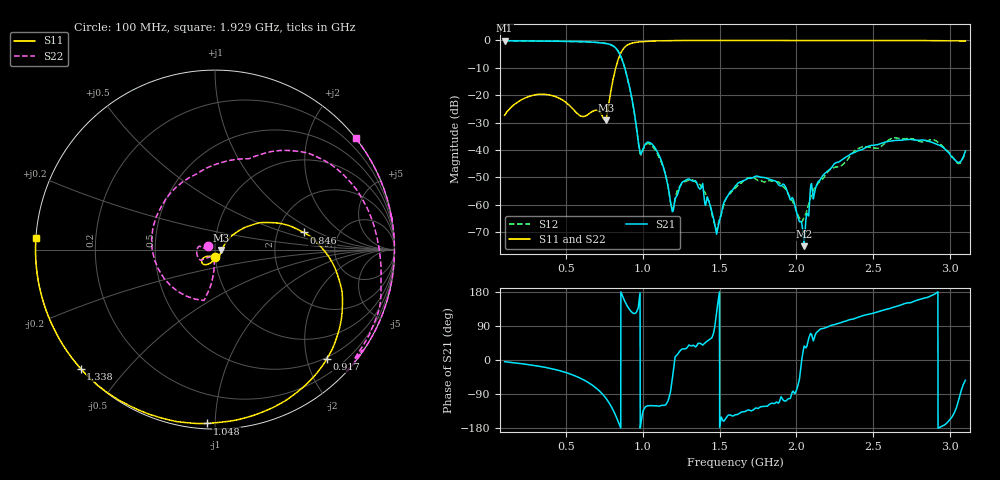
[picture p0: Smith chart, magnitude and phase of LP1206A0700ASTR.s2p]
!	AVX THIN FILM OPERATION
!	LP1206 High Performance Low Pass Filters
!	P/N LP1206A0700ASTR  4 September 2018
!Instrument: 	"HEWLETT PACKARD,8720ES,US39172150,7.62 "
! Created Tue Sep 04 12:40:53 2018
# MHz S db R 50
! freq  dbS11  angS11  dbS21  angS21  dbS12  angS12  dbS22  angS22
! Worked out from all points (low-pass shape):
!   3001 points, 100 MHz to 3.1 GHz, reference 50 ohm
!   highest |S21| = -0.09 dB at 100 MHz (marker M1); lowest = -75.1 dB at 2.05 GHz (marker M2)
!   |S21| within 3 dB of the highest: start of sweep to 828.3 MHz
!   lowest |S11| = -29.2 dB at 760 MHz (marker M3), VSWR 1.07, Z = 53.6 - j0.251 ohm
!   |S11| at or under -10 dB: start of sweep to 823.6 MHz
!   |S22| runs from -29.2 to 0.0 dB; largest |S21 - S12| = 0.024
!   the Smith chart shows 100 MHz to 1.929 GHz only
!   S11 on the Smith chart (normalised r, x): 100 MHz: 1.00, -0.09; 846 MHz: 2.81, +0.72; 917 MHz: 0.47, -2.37; 1.048 GHz: 0.03, -0.95; 1.338 GHz: 0.00, -0.38; 1.929 GHz: -0.00, +0.03
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100  -27.34 -88.4  -0.09 -4.5  -0.09 -4.4  -27.34 153.5
344  -19.63 -131.4  -0.22 -17.9  -0.29 -18.0  -19.63 -158.7
600  -27.69 -112.6  -0.45 -49.4  -0.40 -49.0  -27.69 -111.9
760  -29.17 -3.9  -1.09 -101.0  -1.03 -101.0  -29.17 -94.0
813  -12.48 34.4  -2.26 -137.6  -2.28 -138.1  -12.48 -99.2
846  -5.97 11.0  -4.60 -169.1  -4.52 -171.2  -5.97 80.8
917  -1.20 -44.4  -17.97 131.1  -18.17 131.3  -1.20 17.7
982  -0.51 -73.7  -40.92 177.5  -41.35 -175.0  -0.51 -11.2
1048  -0.27 -92.7  -37.35 -120.3  -37.91 -121.6  -0.27 -18.4
1100  -0.15 -104.2  -41.31 -121.8  -42.02 -122.7  -0.15 -31.9
1191  -0.07 -119.8  -62.22 -52.7  -61.38 -41.0  -0.07 -35.4
1260  -0.02 -129.3  -51.62 29.3  -51.98 34.1  -0.02 -38.1
1338  0.00 -138.5  -51.31 36.2  -51.42 40.0  0.00 -40.9
1481  0.00 -152.3  -70.48 129.5  -69.15 150.0  0.00 -28.6
1600  0.00 -162.1  -53.32 -144.6  -54.08 -138.5  0.00 -18.4
1929  0.00 176.2  -53.49 -108.4  -54.25 -100.0  -0.00 38.3
2050  0.00 169.3  -75.14 37.0  -64.51 44.8  0.00 55.6
2100  0.00 166.4  -53.12 65.3  -56.14 70.2  0.00 68.7
2368  0.00 152.3  -41.07 107.9  -41.02 111.5  0.00 120.5
2600  -0.00 140.5  -36.85 135.0  -36.38 140.2  0.00 -178.2
2832  -0.05 128.6  -36.42 163.4  -36.95 169.1  -0.05 -102.1
3100  -0.22 113.5  -40.39 -53.5  -40.85 -35.5  -0.22 -37.5
